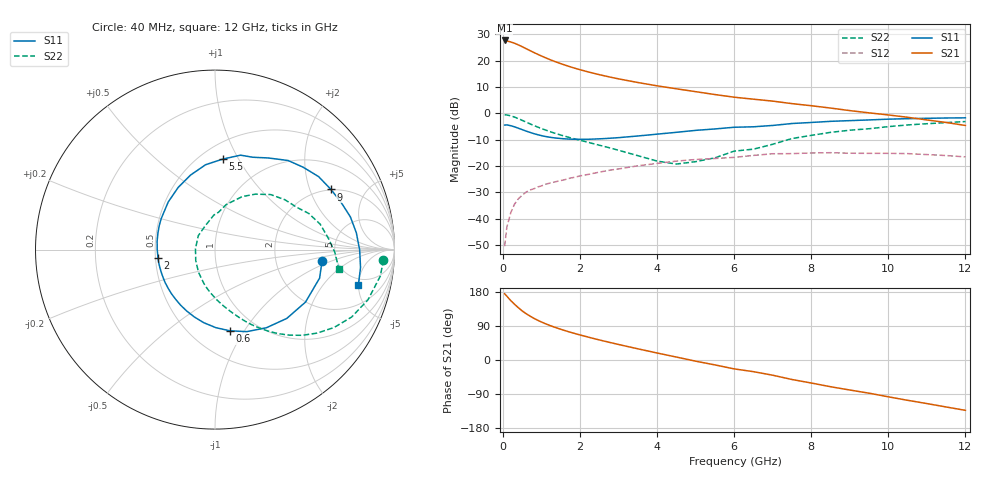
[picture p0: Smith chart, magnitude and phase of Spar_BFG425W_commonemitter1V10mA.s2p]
! Filename: 110bfg425.001
! BFG425W Field C1
! V1=8.540E-001V,V2=1.000E+000V, I1=1.458E-004A, I2=1.002E-002A
# GHz  S  MA  R 50
!  S11  S21  S12  S22
!Freq(GHz)  Mag  Ang  Mag  Ang  Mag  Ang  Mag  Ang
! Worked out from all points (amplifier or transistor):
!   44 points, 40 MHz to 12 GHz, reference 50 ohm
!   highest |S21| = 27.7 dB at 40 MHz (marker M1)
!   |S21| within 3 dB of that: start of sweep to 582 MHz
!   unconditionally stable (mu >= 1): 1.784 GHz to end of sweep
!   at 700 MHz: K = 0.55, MSG = 26.5 dB, |S12| = -29.1 dB
!   at 2.4 GHz: K = 1.12, MAG = 16.7 dB, |S12| = -22.6 dB
!   at 12 GHz: K = 1.39, MAG = 2.3 dB, |S12| = -16.5 dB
!   S11 on the Smith chart (normalised r, x): 40 MHz: 3.83, -0.78; 600 MHz: 0.75, -0.87; 2 GHz: 0.52, -0.05; 5.5 GHz: 0.64, +0.86; 9 GHz: 1.98, +2.82; 12 GHz: 4.03, -4.96
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0.04  0.6 -6.2  24.29 174.9  0.003 75.8  0.94 -3.5
0.1  0.604 -15.3  23.74 168.1  0.007 82.5  0.933 -9.1
0.2  0.583 -30.1  22.72 156.8  0.013 75.2  0.897 -18.2
0.3  0.554 -43.8  21.46 146.9  0.019 69.4  0.849 -26.3
0.4  0.521 -56.8  19.95 137.7  0.024 64.2  0.792 -33.3
0.5  0.49 -68.8  18.43 129.2  0.028 60.0  0.735 -39.3
0.6  0.46 -79.6  16.93 122.1  0.032 56.5  0.682 -44.4
0.8  0.412 -98.7  14.34 110.0  0.037 51.5  0.588 -52.8
0.9  0.393 -106.9  13.25 104.8  0.04 49.8  0.549 -56.3
1.1  0.364 -121.8  11.4 95.7  0.045 47.0  0.483 -62.3
1.3  0.345 -134.9  9.942 87.9  0.049 45.0  0.43 -67.4
1.5  0.333 -146.7  8.79 81.0  0.053 43.2  0.387 -72.0
2  0.321 -171.6  6.746 66.1  0.065 39.1  0.308 -82.9
2.2  0.322 179.7  6.159 60.7  0.069 37.3  0.283 -87.4
3  0.346 149.9  4.524 40.9  0.088 28.8  0.199 -108.1
4.5  0.437 108.2  2.931 7.7  0.124 8.5  0.109 177.7
5.5  0.506 85.2  2.278 -13.0  0.139 -6.5  0.143 112.5
6.5  0.556 67.7  1.86 -30.8  0.159 -18.5  0.209 84.6
8.5  0.706 35.2  1.262 -70.5  0.179 -54.1  0.436 44.7
9  0.728 27.4  1.129 -79.2  0.175 -61.9  0.479 35.4
10.5  0.793 6.8  0.843 -106.3  0.172 -87.5  0.603 13.6
12  0.823 -14.0  0.589 -132.8  0.149 -115.8  0.699 -9.0
